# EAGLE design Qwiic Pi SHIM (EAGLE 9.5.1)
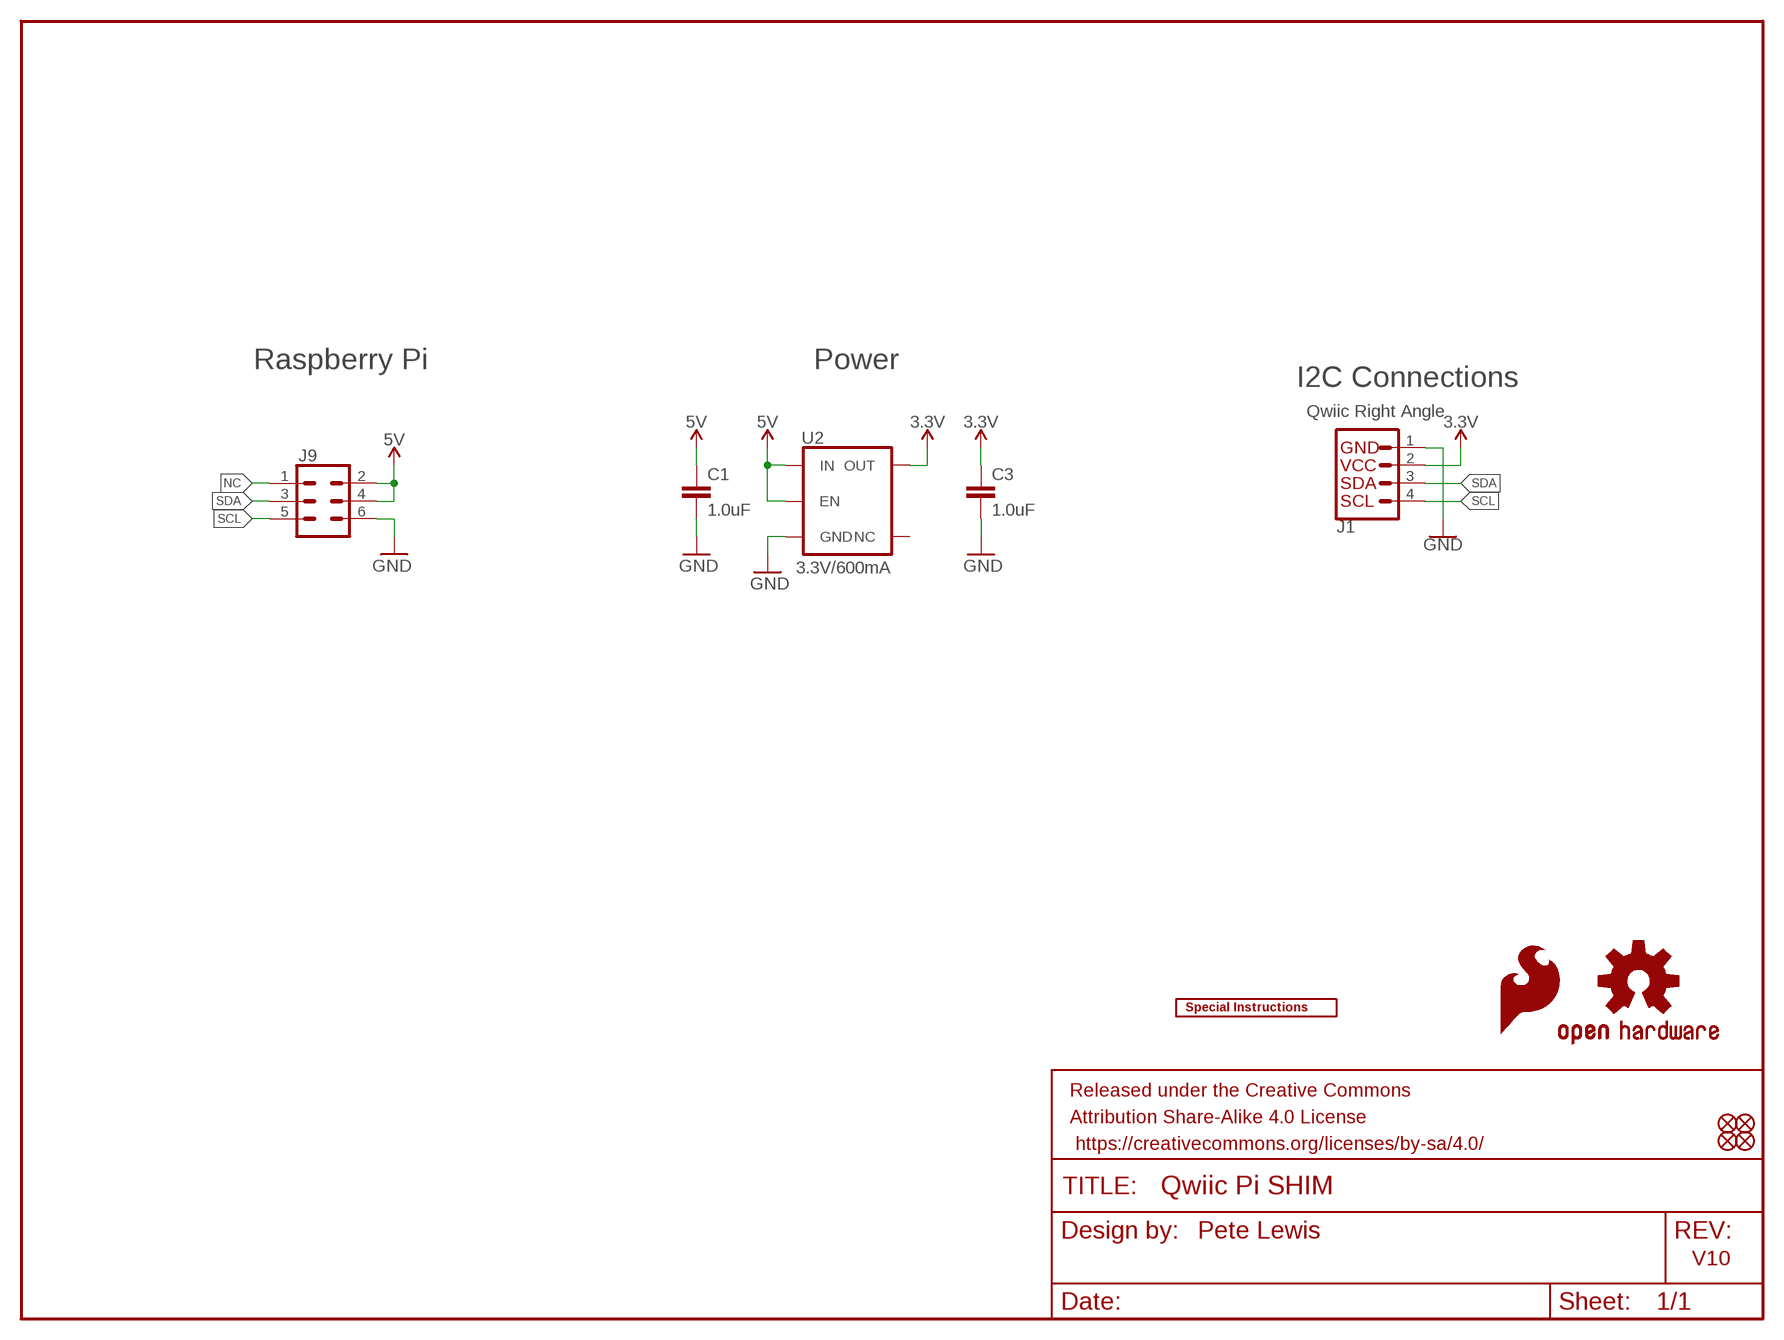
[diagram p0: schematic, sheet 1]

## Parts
C1  1.0uF  1.0UF-0603-16V-10%  [0603]
C3  1.0uF  1.0UF-0603-16V-10%  [0603]
FD1  FIDUCIALUFIDUCIAL  [FIDUCIAL-MICRO]
FD2  FIDUCIALUFIDUCIAL  [FIDUCIAL-MICRO]
FD3  FIDUCIALUFIDUCIAL  [FIDUCIAL-MICRO]
FD4  FIDUCIALUFIDUCIAL  [FIDUCIAL-MICRO]
FRAME1  FRAME-LETTER  [CREATIVE_COMMONS]
J1  Qwiic Right Angle  I2C_STANDARDQWIIC  [1X04_1MM_RA]
J9  SPARKFUN-CONNECTORS_CONN_03X2SINGLE_SLOT-2MILS  [SPARKFUN-CONNECTORS_2X3-NS_PISHIM_LOCKING_SLOTS-2MILS]
LOGO1  OSHW-LOGOMINI  [OSHW-LOGO-MINI]
U2  3.3V/600mA  V_REG_AP2112K-3.3V  [SOT23-5]
U$1  SFE_LOGO_FLAME.1_INCH  [SFE_LOGO_FLAME_.1]
U$4  SPECIAL_INSTRUCTIONS-ORDERING  [ORDERING_INSTRUCTIONS]

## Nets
3.3V: C3.1 J1.2 U2.5(OUT)
5V: C1.1 J9.2 J9.4 U2.1(IN) U2.3(EN)
GND [vcc]: C1.2 C3.2 J1.1 J9.6 U2.2(GND)
NC: J9.1
SCL: J1.4 J9.5
SDA: J1.3 J9.3
Unconnected: U2.4(NC)

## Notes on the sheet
- Raspberry Pi | Power
- I2C Connections
- Pete Lewis
- V10

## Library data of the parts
C1 C3 = SparkFun-Capacitors:1.0UF: 1µF ceramic capacitors; PROD_ID: CAP-00868
FD1-FD4 = SparkFun-Aesthetics:FIDUCIAL: Fiducial Alignment Points
FRAME1 = SparkFun-Aesthetics:FRAME-LETTER: Schematic Frame
J1 = SparkFun-Connectors:I2C_STANDARD: SparkFun I2C Standard Pinout Header SparkFun has standardized on a pinout for all I2C based sensor breakouts. This pinout allows I2C boards to be plugged directly into the headers on Arduino Uno compatible boards, and to be daisy chained easily. Example SparkFun Products: SparkFun Atmospheric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; PROD_ID: CONN-13694
J9 = Qwiic Pi SHIM:SPARKFUN-CONNECTORS_CONN_03X2: Multi connection point. Often used as Generic Header-pin footprint for 0.1 inch spaced/style header connections You can populate with any combo of single row headers, but if you'd like an exact match, check these: Header - 2x3 (Male, 0.1") (PRT-12807) Header - 2x3 (Female, 0.1") (PRT-13010) 2x3 Pin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
LOGO1 = SparkFun-Aesthetics:OSHW-LOGO: Open Source Hardware Logo
U2 = SparkFun-IC-Power:V_REG_AP2112: AP2112 - 600mA CMOS LDO Regulator w/ Enable The AP2112 is CMOS process low dropout linear regulator with enable function, the regulator delivers a guaranteed 600mA (min.) continuous load current. Features Output Voltage Accuracy: ±1.5% Output Current: 600mA (Min.) Foldback Short Current Protection: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; PROD_ID: VREG-12457; VALUE: 3.3V
U$1 = SparkFun-Aesthetics:SFE_LOGO_FLAME: SparkFun Flame Logo
U$4 = SparkFun-Aesthetics:SPECIAL_INSTRUCTIONS: Special Ordering/Production Instructions Alert

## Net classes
0 Default: width 0.178 mm
1 vcc: width 0.178 mm

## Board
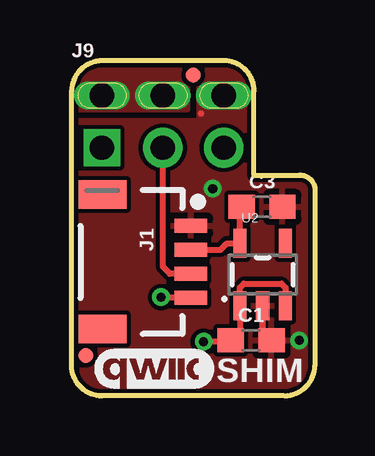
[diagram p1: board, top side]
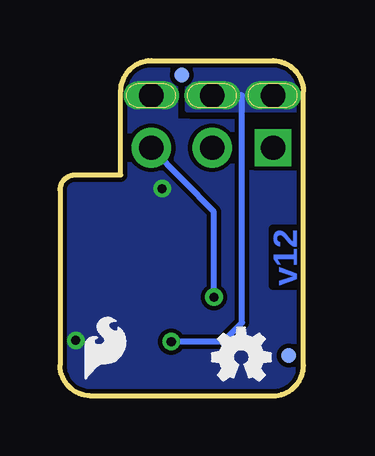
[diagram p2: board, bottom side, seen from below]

Size 10.16 x 13.97 mm. Coordinates in mm from the lower left corner, seen from the top.
Outline: 8.89,0 1.27,0 arc-90 0,1.27 0,12.7 arc-87 1.27,13.97 6.35,13.97 arc-90 7.62,12.7 7.62,9.2 9.53,9.2 arc-90 10.16,8.59 10.16,1.27 arc-87 8.89,0
Copper layers (1*16): Top 0.035mm / dielectric 1.5mm / Bottom 0.035mm
Design rules "SparkFun-2-layer-TIGHT *": minimum track width 7mil, minimum drill 15mil, track to track 7mil, track to pad 7mil, pad to pad 7mil, via to via 7mil, smd to smd 7mil, copper to edge 7mil, drill to drill 7mil, minimum pad ring 2mil, minimum via ring 7mil, stop-mask expansion 4mil, vias tented up to drill 25mil, thermal gap 10mil

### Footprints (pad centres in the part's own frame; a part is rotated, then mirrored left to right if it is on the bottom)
0603 = smd 1.1 x 1: 1 -0.85,0; 2 0.85,0
FIDUCIAL-MICRO = smd 0.635 x 0.635: 1 0,0
1X04_1MM_RA = smd 0.6 x 1.35: 1 -1.5,0; 2 -0.5,0; 3 0.5,0; 4 1.5,0 | smd 1.2 x 2: NC1 2.8,-3.675; NC2 -2.8,-3.675
SPARKFUN-CONNECTORS_2X3-NS_PISHIM_LOCKING_SLOTS-2MILS = drill 1.016 pad 1.524 square: 1 -2.54,-1.092 | drill 1.016 pad 1.168 long: 2 -2.54,1.092; 4 0,1.092; 6 2.54,1.092 | drill 1.016 pad 1.651: 3 0,-1.092; 5 2.54,-1.092
SOT23-5 = smd 0.55 x 1.2: 1 -0.95,-1.3; 2 0,-1.3; 3 0.95,-1.3; 4 0.95,1.3; 5 -0.95,1.3

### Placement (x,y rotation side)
C1  7.49,2.31 0 top
C3  7.95,7.87 0 top
FD1  5.08,13.36 180 top
FD2  0.61,1.68 180 top
FD3  0.61,1.68 0 bottom
FD4  5.08,13.36 0 bottom
FRAME1  not placed on the board
J1  4.98,5.59 270 top
J9  3.81,11.43 0 top
LOGO1  2.59,1.63 0 bottom
U2  7.98,5.05 0 top
U$1  9.42,0.36 0 bottom
U$3  [QWIIC_5MM]  3.43,1.14 0 top
U$4  not placed on the board

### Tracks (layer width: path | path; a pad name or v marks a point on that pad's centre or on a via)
3.3V
  Top 0.254: J1.2 6.21,6.09 6.48,6.36 U2.5 7.03,7.8 C3.1
5V  (via drill 0.38)
  Top 0.254: U2.3 8.93,4.51 8.76,4.67 7.19,4.67 7.03,4.51 U2.1 7.03,2.69 C1.1 6.59,2.26 v5.51,2.26
  Bottom 0.254: v5.51,2.26 3.35,2.26 2.56,3.05 2.56,12.52 J9.4
  pour Top: 4.85,13.97 0,13.97 0,11.91 4.85,11.91
  pour Bottom: 4.85,11.91 0,11.91 0,13.97 4.85,13.97
GND  (via drill 0.38)
  Top 0.254: 5.41,11.76 5.38,11.76 | U2.2 7.98,2.68 C1.2
  other vias: 9.5,2.31 5.89,8.64
  pour Top: 0,11.46 5.33,11.46 5.33,13.97 10.16,13.97 10.16,0 0,0
  pour Bottom: 0.03,11.4 4.8,11.43 5.33,11.43 5.33,13.97 10.16,13.97 10.16,0 0.03,0
SCL  (via drill 0.38)
  Top 0.254: J1.4 3.76,4.09 v3.73,4.12
  Bottom 0.254: J9.5 3.73,7.67 v3.73,4.12
SDA
  Top 0.254: J9.3 3.81,7.62 3.81,5.38 4.11,5.09 J1.3

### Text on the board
Bottom: v12
tPlace: SHIM
tDocu: Pete Lewis | 0.8MM Thickness

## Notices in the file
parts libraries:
SparkFun-Aesthetics: Licensing: CC v3.0 Share-Alike You are welcome to use this library for commercial purposes.
SparkFun-Aesthetics: Released under the Creative Commons Attribution Share-Alike 4.0 License
SparkFun-Aesthetics: https://creativecommons.org/licenses/by-sa/4.0
